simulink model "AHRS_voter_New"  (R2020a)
settings: Solver=FixedStepDiscrete  StartTime=0.0  StopTime=10.0  FixedStep=0.01  RelTol=1e-3  EnableMultiTasking=on
model workspace (MAT data in the model file):
  Ts : Simulink.Parameter (value not decoded)
libraries: simulink x1

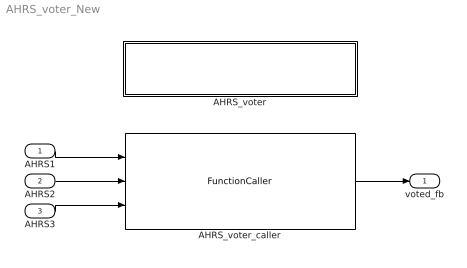
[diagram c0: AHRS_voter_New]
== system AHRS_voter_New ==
  AHRS1 : Inport  OutDataTypeStr=Bus: AHRS_Bus
  AHRS2 : Inport  Port=2  OutDataTypeStr=Bus: AHRS_Bus
  AHRS3 : Inport  Port=3  OutDataTypeStr=Bus: AHRS_Bus
  AHRS_voter : Subsystem  TreatAsAtomicUnit=on
  AHRS_voter_caller : FunctionCaller  FunctionPrototype=voted_fb = AHRS_voter(AHRS1,AHRS2,AHRS3)
  voted_fb : Outport
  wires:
  AHRS1/1 -> AHRS_voter_caller/1
  AHRS2/1 -> AHRS_voter_caller/2
  AHRS3/1 -> AHRS_voter_caller/3
  AHRS_voter_caller/1 -> voted_fb/1

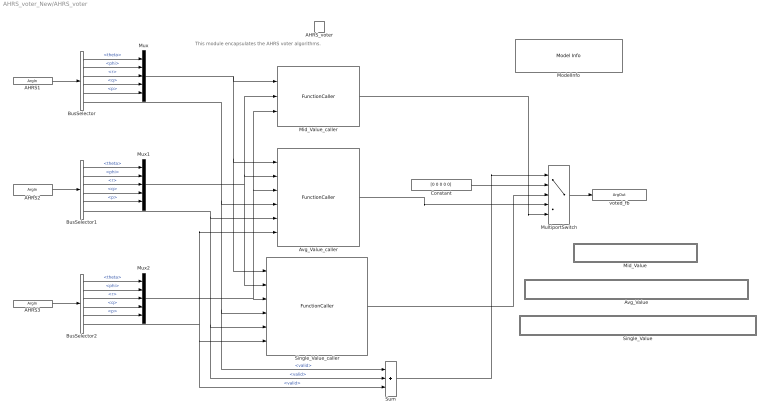
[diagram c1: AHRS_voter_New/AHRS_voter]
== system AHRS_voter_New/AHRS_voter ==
  note: This module encapsulates the AHRS voter algorithms.
  AHRS_voter : TriggerPort  TriggerType=function-call  IsSimulinkFunction=on  FunctionName=AHRS_voter  FunctionVisibility=scoped  VariantControl=Variant  PortDimensions=1
  Avg_Value : Subsystem  TreatAsAtomicUnit=on  RTWFcnName=Avg_Value
  Avg_Value_caller : FunctionCaller  FunctionPrototype=Avg_Value = Avg_Value(AHRS1,AHRS2,AHRS3,AHRS1_Valid,AHRS2_Valid,AHRS3_Valid)
  BusSelector : BusSelector  OutputSignals=theta,phi,r,q,p,valid
  BusSelector1 : BusSelector  OutputSignals=theta,phi,r,q,p,valid
  BusSelector2 : BusSelector  OutputSignals=theta,phi,r,q,p,valid
  Constant : Constant  Value=[0 0 0 0 0]
  Mid_Value : Subsystem  TreatAsAtomicUnit=on  RTWFcnName=Mid_Value
  Mid_Value_caller : FunctionCaller  FunctionPrototype=Mid_Value = Mid_Value(AHRS1,AHRS2,AHRS3)
  ModelInfo : simulink/Model-Wide Utilities/Model Info  Frame=on  DisplayStringWithTags=|  HorizontalTextAlignment=Center  LeftAlignmentValue=0.5
      | Model Name: %<ModelName>
      | Model Version: %<ModelVersion>
      | Last Modified: %<LastModificationDate>
      | 
      | Copyright 2016 The MathWorks, Inc.
  MultiportSwitch : MultiPortSwitch  DataPortOrder=Zero-based contiguous  Inputs=4  DiagnosticForDefault=None  zeroidx=on
  Mux : Mux  Inputs=5
  Mux1 : Mux  Inputs=5
  Mux2 : Mux  Inputs=5
  Single_Value : Subsystem  TreatAsAtomicUnit=on  RTWFcnName=Single_Value
  Single_Value_caller : FunctionCaller  FunctionPrototype=Single_Value = Single_Value(AHRS1,AHRS2,AHRS3,AHRS1_Valid,AHRS2_Valid,AHRS3_Valid)
  Sum : Sum  Inputs=+++  OutDataTypeStr=uint32
  AHRS1 : ArgIn  OutDataTypeStr=Bus: AHRS_Bus  ArgumentName=AHRS1
  AHRS2 : ArgIn  Port=2  OutDataTypeStr=Bus: AHRS_Bus  ArgumentName=AHRS2
  AHRS3 : ArgIn  Port=3  OutDataTypeStr=Bus: AHRS_Bus  ArgumentName=AHRS3
  voted_fb : ArgOut  PortDimensions=5  ArgumentName=voted_fb
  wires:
  BusSelector2/5 -> Mux2/5  "<p>"
  Mux2/1 -> Avg_Value_caller/3, Mid_Value_caller/3, Single_Value_caller/3
  BusSelector/4 -> Mux/4  "<q>"
  BusSelector2/1 -> Mux2/1  "<theta>"
  BusSelector/2 -> Mux/2  "<phi>"
  BusSelector2/2 -> Mux2/2  "<phi>"
  BusSelector2/3 -> Mux2/3  "<r>"
  BusSelector1/2 -> Mux1/2  "<phi>"
  Sum/1 -> MultiportSwitch/1
  BusSelector1/4 -> Mux1/4  "<q>"
  Constant/1 -> MultiportSwitch/2
  BusSelector2/4 -> Mux2/4  "<q>"
  BusSelector2/6 -> Sum/3, Single_Value_caller/6, Avg_Value_caller/6  "<valid>"
  BusSelector/6 -> Sum/1, Single_Value_caller/4, Avg_Value_caller/4  "<valid>"
  BusSelector1/3 -> Mux1/3  "<r>"
  BusSelector/1 -> Mux/1  "<theta>"
  Mux/1 -> Mid_Value_caller/1, Single_Value_caller/1, Avg_Value_caller/1
  BusSelector/3 -> Mux/3  "<r>"
  Single_Value_caller/1 -> MultiportSwitch/3
  BusSelector1/1 -> Mux1/1  "<theta>"
  BusSelector1/5 -> Mux1/5  "<p>"
  Mux1/1 -> Single_Value_caller/2, Avg_Value_caller/2, Mid_Value_caller/2
  BusSelector/5 -> Mux/5  "<p>"
  MultiportSwitch/1 -> voted_fb/1
  Mid_Value_caller/1 -> MultiportSwitch/5
  Avg_Value_caller/1 -> MultiportSwitch/4
  BusSelector1/6 -> Sum/2, Single_Value_caller/5, Avg_Value_caller/5  "<valid>"
  AHRS1/1 -> BusSelector/1
  AHRS2/1 -> BusSelector1/1
  AHRS3/1 -> BusSelector2/1

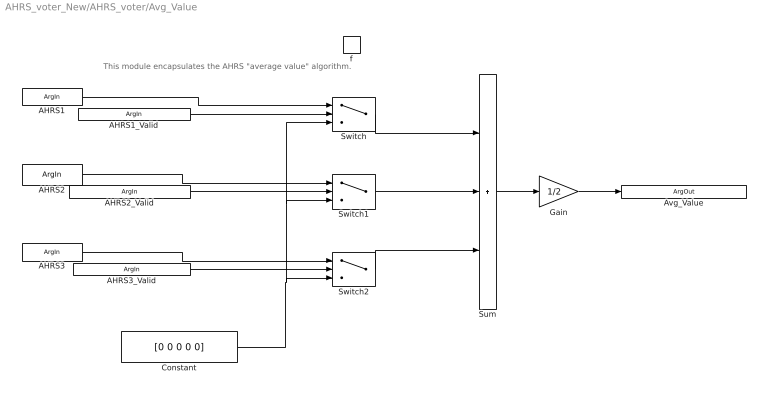
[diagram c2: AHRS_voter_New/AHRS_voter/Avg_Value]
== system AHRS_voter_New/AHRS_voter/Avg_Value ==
  note: This module encapsulates the AHRS "average value" algorithm.
  f : TriggerPort  TriggerType=function-call  IsSimulinkFunction=on  FunctionName=Avg_Value  FunctionVisibility=scoped  VariantControl=Variant  PortDimensions=1
  Constant : Constant  Value=[0 0 0 0 0]
  Gain : Gain  Gain=1/2
  Sum : Sum  Inputs=+++
  Switch : Switch  Criteria=u2 ~= 0
  Switch1 : Switch  Criteria=u2 ~= 0
  Switch2 : Switch  Criteria=u2 ~= 0
  AHRS1 : ArgIn  PortDimensions=5  ArgumentName=AHRS1
  AHRS2 : ArgIn  Port=2  PortDimensions=5  ArgumentName=AHRS2
  AHRS3 : ArgIn  Port=3  PortDimensions=5  ArgumentName=AHRS3
  AHRS1_Valid : ArgIn  Port=4  OutDataTypeStr=boolean  ArgumentName=AHRS1_Valid
  AHRS2_Valid : ArgIn  Port=5  OutDataTypeStr=boolean  ArgumentName=AHRS2_Valid
  AHRS3_Valid : ArgIn  Port=6  OutDataTypeStr=boolean  ArgumentName=AHRS3_Valid
  Avg_Value : ArgOut  PortDimensions=5  ArgumentName=Avg_Value
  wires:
  Gain/1 -> Avg_Value/1
  Sum/1 -> Gain/1
  AHRS1_Valid/1 -> Switch/2
  AHRS1/1 -> Switch/1
  Switch/1 -> Sum/1
  Switch1/1 -> Sum/2
  Switch2/1 -> Sum/3
  AHRS2_Valid/1 -> Switch1/2
  AHRS3_Valid/1 -> Switch2/2
  AHRS2/1 -> Switch1/1
  AHRS3/1 -> Switch2/1
  Constant/1 -> Switch/3, Switch1/3, Switch2/3

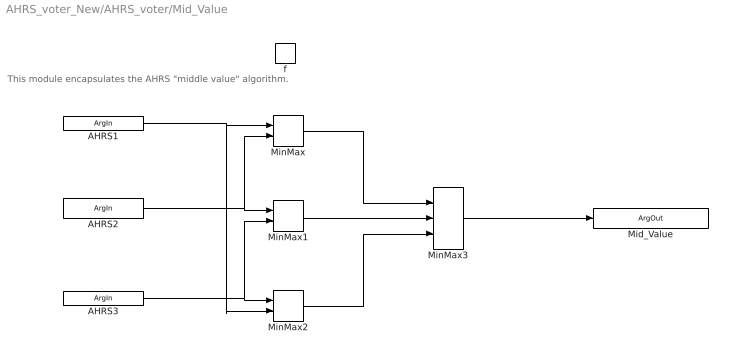
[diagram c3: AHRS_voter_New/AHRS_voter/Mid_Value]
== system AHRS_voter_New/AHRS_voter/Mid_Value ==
  note: This module encapsulates the AHRS "middle value" algorithm.
  f : TriggerPort  TriggerType=function-call  IsSimulinkFunction=on  FunctionName=Mid_Value  FunctionVisibility=scoped  VariantControl=Variant  PortDimensions=1
  MinMax : MinMax  Inputs=2
  MinMax1 : MinMax  Inputs=2
  MinMax2 : MinMax  Inputs=2
  MinMax3 : MinMax  Function=max  Inputs=3
  AHRS1 : ArgIn  PortDimensions=5  ArgumentName=AHRS1
  AHRS2 : ArgIn  Port=2  PortDimensions=5  ArgumentName=AHRS2
  AHRS3 : ArgIn  Port=3  PortDimensions=5  ArgumentName=AHRS3
  Mid_Value : ArgOut  PortDimensions=5  ArgumentName=Mid_Value
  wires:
  AHRS1/1 -> MinMax2/2, MinMax/1
  AHRS3/1 -> MinMax1/2, MinMax2/1
  AHRS2/1 -> MinMax/2, MinMax1/1
  MinMax1/1 -> MinMax3/2
  MinMax/1 -> MinMax3/1
  MinMax2/1 -> MinMax3/3
  MinMax3/1 -> Mid_Value/1

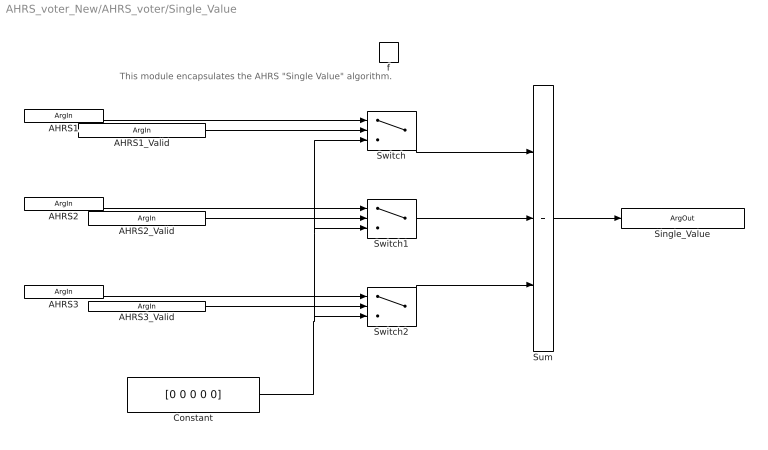
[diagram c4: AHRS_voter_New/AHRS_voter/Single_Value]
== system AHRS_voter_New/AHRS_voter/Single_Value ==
  note: This module encapsulates the AHRS "Single Value" algorithm.
  f : TriggerPort  TriggerType=function-call  IsSimulinkFunction=on  FunctionName=Single_Value  FunctionVisibility=scoped  VariantControl=Variant  PortDimensions=1
  Constant : Constant  Value=[0 0 0 0 0]
  Sum : Sum  Inputs=+++
  Switch : Switch  Criteria=u2 ~= 0
  Switch1 : Switch  Criteria=u2 ~= 0
  Switch2 : Switch  Criteria=u2 ~= 0
  AHRS1 : ArgIn  PortDimensions=5  ArgumentName=AHRS1
  AHRS2 : ArgIn  Port=2  PortDimensions=5  ArgumentName=AHRS2
  AHRS3 : ArgIn  Port=3  PortDimensions=5  ArgumentName=AHRS3
  AHRS1_Valid : ArgIn  Port=4  OutDataTypeStr=boolean  ArgumentName=AHRS1_Valid
  AHRS2_Valid : ArgIn  Port=5  OutDataTypeStr=boolean  ArgumentName=AHRS2_Valid
  AHRS3_Valid : ArgIn  Port=6  OutDataTypeStr=boolean  ArgumentName=AHRS3_Valid
  Single_Value : ArgOut  PortDimensions=5  ArgumentName=Single_Value
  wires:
  Constant/1 -> Switch2/3, Switch1/3, Switch/3
  AHRS3/1 -> Switch2/1
  AHRS2/1 -> Switch1/1
  AHRS3_Valid/1 -> Switch2/2
  AHRS2_Valid/1 -> Switch1/2
  Switch2/1 -> Sum/3
  Switch1/1 -> Sum/2
  Switch/1 -> Sum/1
  AHRS1/1 -> Switch/1
  AHRS1_Valid/1 -> Switch/2
  Sum/1 -> Single_Value/1
